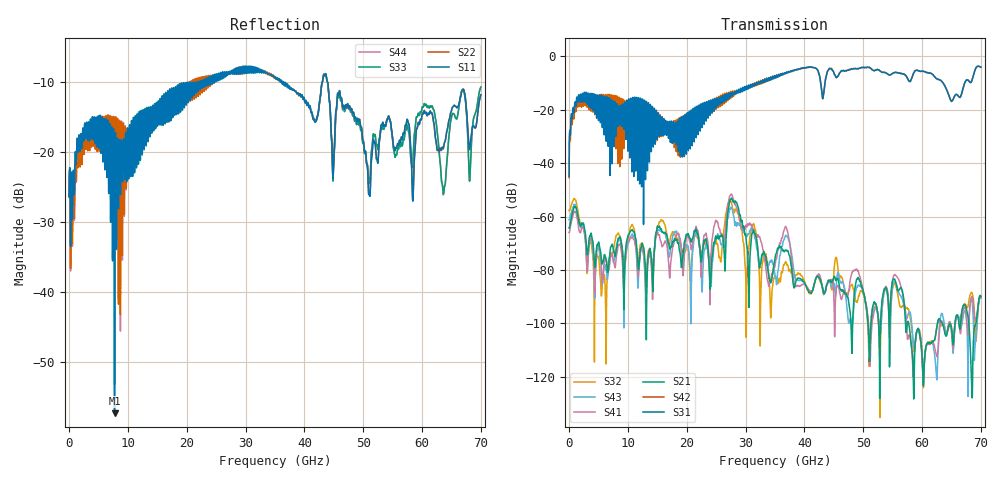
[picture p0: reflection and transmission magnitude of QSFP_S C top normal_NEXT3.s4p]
! AWR Design Environment (8415) Tue Jan 08 11:56:37 2019
! Document = 'QSFP Channel_S'
! nPorts: 4, nXvals: 7001
# HZ S DB R 50
!Freq DBS11 AngS11 DBS12 AngS12 DBS13 AngS13 DBS14 AngS14
!	DBS21 AngS21 DBS22 AngS22 DBS23 AngS23 DBS24 AngS24
!	DBS31 AngS31 DBS32 AngS32 DBS33 AngS33 DBS34 AngS34
!	DBS41 AngS41 DBS42 AngS42 DBS43 AngS43 DBS44 AngS44
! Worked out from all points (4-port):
!   7000 points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, 10 MHz to 70 GHz, reference 50 ohm
!   strongest paths, dB at 10 MHz, 17.51 GHz, 35.01 GHz, 52.51 GHz, 70 GHz:
!     S31: -44.9, -30.3, -7.3, -5.0, -4.0
!     S42: -45.5, -27.8, -7.4, -5.0, -4.0
!     S21: -64.3, -70.5, -75.7, -97.1, -89.8
!     S41: -65.9, -73.1, -78.4, -96.6, -90.2
!     S43: -61.2, -68.5, -81.9, -96.4, -90.6
!     S32: -57.7, -66.2, -82.6, -97.0, -90.3
!   lowest |S11| = -57.3 dB at 7.73 GHz (marker M1), VSWR 1.00, Z = 49.9 + j0.127 ohm
!   |S11| at or under -10 dB: start of sweep to 20.42 GHz; 36.48 GHz to 43.04 GHz (6.553 GHz wide, 16.5 % of centre); 43.96 GHz to end of sweep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
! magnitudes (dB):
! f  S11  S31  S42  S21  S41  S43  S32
! 10 MHz  -26.3  -44.9  -45.5  -64.3  -65.9  -61.2  -57.7
! 1.63 GHz  -18.3  -14.4  -15.6  -61.6  -64.5  -61.8  -59.8
! 7.73 GHz  -57.3  -18.1  -16.5  -73.9  -78.3  -75.8  -70.1
! 24.05 GHz  -9.6  -17.3  -18.1  -85.8  -79.3  -84.0  -75.7
! 27.55 GHz  -8.7  -14.1  -14.2  -53.2  -51.6  -56.5  -54.5
! 33.83 GHz  -8.8  -9.0  -8.9  -80.3  -84.7  -78.2  -79.1
! 70 GHz  -11.8  -4.0  -4.0  -89.8  -90.2  -90.6  -90.3
